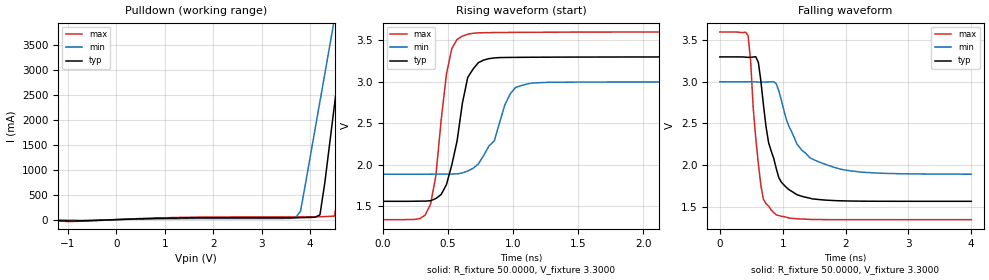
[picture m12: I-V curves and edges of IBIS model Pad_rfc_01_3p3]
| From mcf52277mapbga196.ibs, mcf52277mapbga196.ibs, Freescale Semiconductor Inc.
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|   Model Pad_rfc_01_3p3
[Model]   Pad_rfc_01_3p3
Model_type   Open_drain
Polarity   Non-Inverting
Enable   Active-High
Vmeas =   1.6500V
C_comp   1.7450pF   1.6200pF   1.8900pF
[Temperature Range]   25.0000   0.1500k   -40.0000
[Voltage Range]   3.3000V   3.0000V   3.6000V
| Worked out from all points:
|   slope of the pulldown table from 0 to 0.495 V, typ, clamps not added: 30.6 ohm
|   rising waveform, R_fixture 50.0000, V_fixture 3.3000: 20-80 % time 124ps typ, 181ps min, 97.6ps max; typ from 1.56 V to 3.3 V
|   falling waveform, R_fixture 50.0000, V_fixture 3.3000: 20-80 % time 254ps typ, 423ps min, 149ps max; typ from 3.3 V to 1.56 V
[Pulldown]
| voltage   I(typ)   I(min)   I(max)
-3.3V     -390uA     -280uA     -450uA
-1V       -25.77mA   -11.5mA    -37.44mA
1.3V      32.05mA    19.89mA    44.41mA
3.7V      39.17mA    37.43mA    55.33mA
3.8V      39.59mA    171.6mA    55.46mA
4.2V      96.59mA    2.369A     57.73mA
4.3V      736.9mA    2.923A     60.8mA
4.5V      2.305A     4.03A      71.43mA
4.7V      3.874A     5.139A     1.283A
4.9V      5.445A     6.248A     3.288A
5.1V      7.018A     7.359A     5.296A
6.6V      18.83A     15.7A      20.38A
[Ramp]
| variable   typ   min   max
dV/dt_r   1.0424/0.1220n   0.6665/0.1792n   1.3551/98.2545p
dV/dt_f   1.0425/0.2576n   0.6665/0.4201n   1.3552/0.1566n
R_load = 50.0000
[Rising Waveform]
R_fixture = 50.0000
V_fixture = 3.3000
V_fixture_min = 3.0000
V_fixture_max = 3.6000
| time   V(typ)   V(min)   V(max)
0s        1.562V     1.889V     1.341V
367.3ps   1.569V     1.889V     1.526V
408.2ps   1.596V     1.889V     1.866V
489.8ps   1.763V     1.89V      3.094V
530.6ps   1.998V     1.89V      3.398V
612.2ps   2.744V     1.903V     3.55V
734.7ps   3.23V      2.011V     3.589V
979.6ps   3.294V     2.856V     3.595V
1.143ns   3.296V     2.985V     3.596V
4ns       3.3V       3V         3.6V
[Falling Waveform]
R_fixture = 50.0000
V_fixture = 3.3000
V_fixture_min = 3.0000
V_fixture_max = 3.6000
| time   V(typ)   V(min)   V(max)
0s        3.3V       3V         3.6V
449ps     3.295V     3V         3.557V
489.8ps   3.295V     3V         3.256V
571.4ps   3.302V     2.999V     2.322V
653.1ps   3.009V     2.997V     1.751V
775.5ps   2.269V     2.999V     1.505V
898ps     1.956V     2.976V     1.4V
1.225ns   1.643V     2.254V     1.353V
1.51ns    1.589V     2.058V     1.344V
4ns       1.562V     1.889V     1.341V
